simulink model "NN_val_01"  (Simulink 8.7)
settings: Solver=ode45  StartTime=0.0  StopTime=1000  RelTol=1e-3
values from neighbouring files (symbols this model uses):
  Ts = 0.05    [init_model.m]
libraries: neural x26

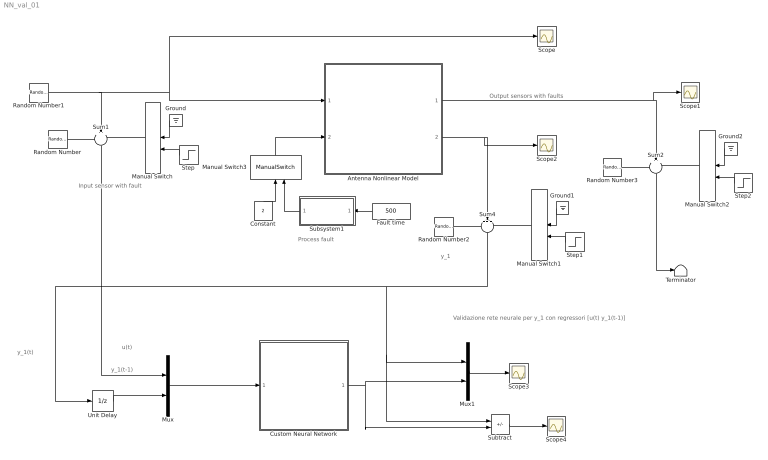
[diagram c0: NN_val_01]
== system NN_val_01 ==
  note: Validazione rete neurale per y_1 con regressori [u(t) y_1(t-1)]
  note: y_1(t)
  note: y_1(t-1)
  note: y_1
  note: u(t)
  note: Output sensors with faults
  note: Process fault
  note: Input sensor with fault
  Antenna Nonlinear Model : Subsystem
  Constant : Constant  Value=2
  Custom Neural Network : Subsystem
  Fault time : Constant  Value=500
  Ground : Ground
  Ground1 : Ground
  Ground2 : Ground
  Manual Switch{,1..3} (4 alike) : ManualSwitch
  Mux : Mux  Inputs=2
  Mux1 : Mux  Inputs=2
  Random Number : RandomNumber  Variance=0.0001  Seed=1  SampleTime=Ts
  Random Number1 : RandomNumber  Variance=0.1  SampleTime=10
  Random Number2 : RandomNumber  Variance=0.00001  Seed=2  SampleTime=Ts
  Random Number3 : RandomNumber  Variance=0.00001  Seed=3  SampleTime=Ts
  Scope{,1..4} (5 alike) : Scope
  Step : Step  Time=500  SampleTime=0
  Step1 : Step  Time=500  SampleTime=0
  Step2 : Step  Time=500  SampleTime=0
  Subsystem1 : Subsystem
  Subtract : Sum  Inputs=+-
  Sum1 : Sum  Inputs=+++  SaturateOnIntegerOverflow=on
  Sum2 : Sum  Inputs=+++  SaturateOnIntegerOverflow=on
  Sum4 : Sum  Inputs=+++  SaturateOnIntegerOverflow=on
  Terminator : Terminator
  Unit Delay : UnitDelay  SampleTime=Ts  HasFrameUpgradeWarning=on
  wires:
  Random Number1/1 -> Scope/1, Antenna Nonlinear Model/1(force), Sum1/2
  Random Number/1 -> Sum1/1
  Manual Switch/1 -> Sum1/3
  Sum1/1 -> Mux/1
  Ground/1 -> Manual Switch/1
  Step/1 -> Manual Switch/2
  Random Number2/1 -> Sum4/1
  Ground1/1 -> Manual Switch1/1
  Manual Switch1/1 -> Sum4/3
  Step1/1 -> Manual Switch1/2
  Antenna Nonlinear Model/2(velocity) -> Sum4/2, Scope2/1
  Random Number3/1 -> Sum2/1
  Ground2/1 -> Manual Switch2/1
  Manual Switch2/1 -> Sum2/3
  Step2/1 -> Manual Switch2/2
  Antenna Nonlinear Model/1(angle) -> Sum2/2, Scope1/1
  Sum2/1 -> Terminator/1
  Fault time/1 -> Subsystem1/1(Fault time)
  Subsystem1/1(Fault) -> Manual Switch3/2
  Manual Switch3/1 -> Antenna Nonlinear Model/2(drag)
  Constant/1 -> Manual Switch3/1
  Mux/1 -> Custom Neural Network/1(Input)
  Sum4/1 -> Subtract/1, Mux1/1, Unit Delay/1
  Unit Delay/1 -> Mux/2
  Custom Neural Network/1(Output) -> Subtract/2, Mux1/2
  Mux1/1 -> Scope3/1
  Subtract/1 -> Scope4/1

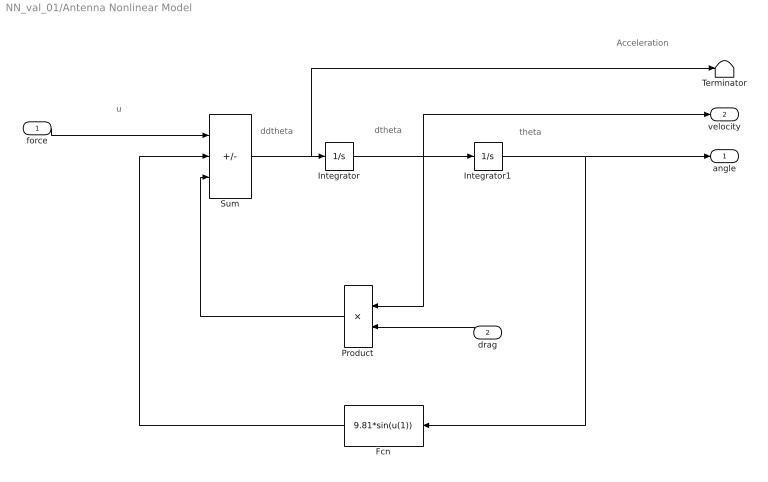
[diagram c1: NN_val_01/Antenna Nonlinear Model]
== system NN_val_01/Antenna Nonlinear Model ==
  note: Acceleration
  note: ddtheta
  note: dtheta
  note: theta
  note: u
  force : Inport
  drag : Inport  Port=2
  Fcn : Fcn  Expr=9.81*sin(u(1))
  Integrator : Integrator
  Integrator1 : Integrator  InitialCondition=(pi/180)*90
  Product : Product
  Sum : Sum  Inputs=+--  SaturateOnIntegerOverflow=on
  Terminator : Terminator
  angle : Outport
  velocity : Outport  Port=2
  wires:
  Sum/1 -> Terminator/1, Integrator/1
  Integrator/1 -> Product/1, Integrator1/1, velocity/1
  Integrator1/1 -> angle/1, Fcn/1
  Fcn/1 -> Sum/2
  Product/1 -> Sum/3
  force/1 -> Sum/1
  drag/1 -> Product/2

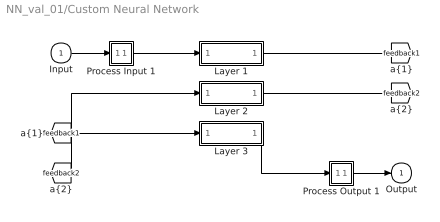
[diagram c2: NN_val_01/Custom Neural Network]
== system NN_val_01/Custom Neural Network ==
  Input : Inport  PortDimensions=2  SampleTime=0.05
  Layer 1 : Subsystem
  Layer 2 : Subsystem
  Layer 3 : Subsystem
  Process Input 1 : Subsystem
  Process Output 1 : Subsystem
  Output : Outport  InitialOutput=0
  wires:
  Input/1 -> Process Input 1/1(x)
  Process Output 1/1(y) -> Output/1
  Process Input 1/1(p) -> Layer 1/1("p{1}")
  Layer 1/1("a{1}") -> [feedback1]
  [feedback1] -> Layer 2/1("a{1} ")
  Layer 2/1("a{2}") -> [feedback2]
  [feedback2] -> Layer 3/1("a{2} ")
  Layer 3/1("a{3}") -> Process Output 1/1(a)

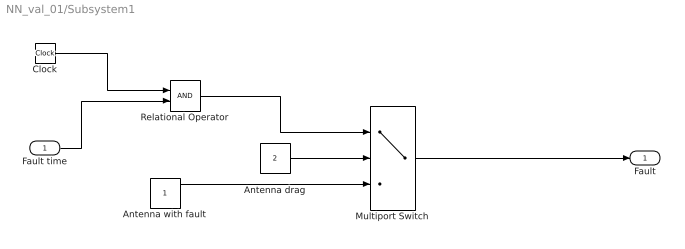
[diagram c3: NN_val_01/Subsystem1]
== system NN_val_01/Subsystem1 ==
  Fault time : Inport
  Antenna drag : Constant  Value=2
  Antenna with fault : Constant
  Clock : Clock
  Multiport Switch : MultiPortSwitch  DataPortOrder=Zero-based contiguous  Inputs=2  zeroidx=on
  Relational Operator : RelationalOperator  OutDataTypeStr=boolean
  Fault : Outport
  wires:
  Clock/1 -> Relational Operator/1
  Fault time/1 -> Relational Operator/2
  Antenna drag/1 -> Multiport Switch/2
  Relational Operator/1 -> Multiport Switch/1
  Multiport Switch/1 -> Fault/1
  Antenna with fault/1 -> Multiport Switch/3

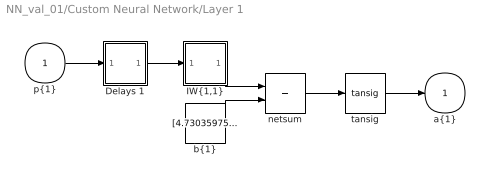
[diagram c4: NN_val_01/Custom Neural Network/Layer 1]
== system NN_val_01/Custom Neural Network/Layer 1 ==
  "p{1}" : Inport  PortDimensions=2  SampleTime=0.05
  Delays 1 : Subsystem
  "IW{1,1}" : Subsystem
  "b{1}" : Constant  Value=[4.73035975157952837122365963296033442020416259765625;1.92318223342469263315024363691918551921844482421875;0.67941730006991007950745142807136289775371551513671875;-0.8082785614923551076316243779729120433330535888671875;0.9412319551905510284228739692480303347110748291015625;-1.385422663696747491712812916375696659088134765625;4.98532785766653585568519702064804732799530029296875]
  netsum : Sum  Inputs=2  InputSameDT=on  SaturateOnIntegerOverflow=on
  tansig : neural/Transfer Functions/tansig
  "a{1}" : Outport  InitialOutput=[0;0;0;0;0;0;0]
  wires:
  "p{1}"/1 -> Delays 1/1("p{1}")
  Delays 1/1("pd{1,1}") -> "IW{1,1}"/1("pd{1,1}")
  "IW{1,1}"/1("iz{1,1}") -> netsum/1
  "b{1}"/1 -> netsum/2
  netsum/1 -> tansig/1
  tansig/1 -> "a{1}"/1

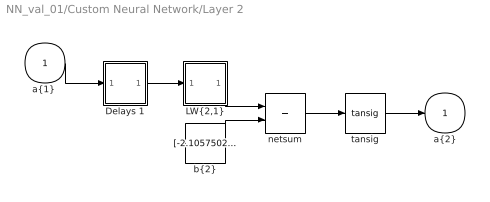
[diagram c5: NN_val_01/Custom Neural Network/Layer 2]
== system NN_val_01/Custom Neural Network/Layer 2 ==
  "a{1} " : Inport  PortDimensions=7  SampleTime=0.05
  Delays 1 : Subsystem
  "LW{2,1}" : Subsystem
  "b{2}" : Constant  Value=[-2.10575022370540665406224434264004230499267578125;-1.740826910029001250990177140920422971248626708984375;1.2556473118148903100887991968193091452121734619140625;-1.26621592229308976840229661320336163043975830078125;-0.83947473433330987990785843066987581551074981689453125;-0.6627922058413020511835611614515073597431182861328125;-0.428254180079056190333375297996099106967449188232421875;-0.1999065764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
  netsum : Sum  Inputs=2  InputSameDT=on  SaturateOnIntegerOverflow=on
  tansig : neural/Transfer Functions/tansig
  "a{2}" : Outport  InitialOutput=[0;0;0;0;0;0;0;0;0;0;0;0;0;0;0]
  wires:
  "a{1} "/1 -> Delays 1/1("p{2}")
  Delays 1/1("pd{2,1}") -> "LW{2,1}"/1("ad{2,1}")
  "LW{2,1}"/1("lz{2,1}") -> netsum/1
  "b{2}"/1 -> netsum/2
  netsum/1 -> tansig/1
  tansig/1 -> "a{2}"/1

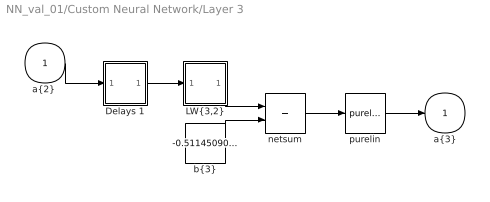
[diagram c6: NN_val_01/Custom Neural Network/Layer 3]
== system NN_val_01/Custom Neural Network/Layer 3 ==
  "a{2} " : Inport  PortDimensions=15  SampleTime=0.05
  Delays 1 : Subsystem
  "LW{3,2}" : Subsystem
  "b{3}" : Constant  Value=-0.51145090309600893530017629018402658402919769287109375
  netsum : Sum  Inputs=2  InputSameDT=on  SaturateOnIntegerOverflow=on
  purelin : neural/Transfer Functions/purelin
  "a{3}" : Outport  InitialOutput=0
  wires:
  "a{2} "/1 -> Delays 1/1("p{3}")
  Delays 1/1("pd{3,2}") -> "LW{3,2}"/1("ad{3,2}")
  "LW{3,2}"/1("lz{3,2}") -> netsum/1
  "b{3}"/1 -> netsum/2
  netsum/1 -> purelin/1
  purelin/1 -> "a{3}"/1

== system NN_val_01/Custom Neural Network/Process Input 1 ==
  x : Inport  PortDimensions=2  SampleTime=0.05
  p : Outport  PortDimensions=2  SampleTime=0.05
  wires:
  x/1 -> p/1

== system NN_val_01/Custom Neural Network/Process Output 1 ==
  a : Inport  PortDimensions=1  SampleTime=0.05
  y : Outport  PortDimensions=1  SampleTime=0.05
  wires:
  a/1 -> y/1

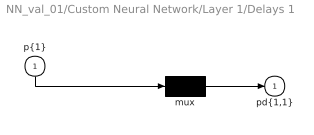
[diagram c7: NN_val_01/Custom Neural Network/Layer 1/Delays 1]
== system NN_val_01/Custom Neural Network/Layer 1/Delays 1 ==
  "p{1}" : Inport  PortDimensions=2  SampleTime=0.05
  mux : Mux  Inputs=1
  "pd{1,1}" : Outport
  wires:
  "p{1}"/1 -> mux/1
  mux/1 -> "pd{1,1}"/1

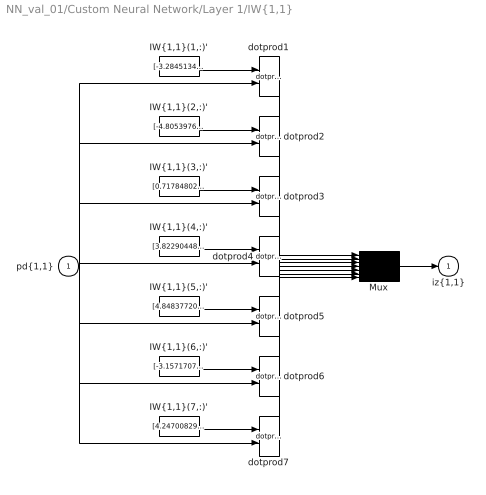
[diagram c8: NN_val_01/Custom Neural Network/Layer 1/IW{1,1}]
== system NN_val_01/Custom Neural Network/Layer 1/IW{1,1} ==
  "pd{1,1}" : Inport  PortDimensions=2  SampleTime=0.05
  "IW{1,1}(1,:)'" : Constant  Value=[-3.28451341394441076459997930214740335941314697265625;1.51253223920159829418707886361517012119293212890625]
  "IW{1,1}(2,:)'" : Constant  Value=[-4.8053976456978002573805497377179563045501708984375;-0.2265032205568367762449355495846248231828212738037109375]
  "IW{1,1}(3,:)'" : Constant  Value=[0.71784802946217818320207015858613885939121246337890625;1.456825343686549700805699103511869907379150390625]
  "IW{1,1}(4,:)'" : Constant  Value=[3.822904484041890871282021180377341806888580322265625;-1.11503162371019204357480703038163483142852783203125]
  "IW{1,1}(5,:)'" : Constant  Value=[4.848377202356548565376215265132486820220947265625;-0.284036485298596985682451077082077972590923309326171875]
  "IW{1,1}(6,:)'" : Constant  Value=[-3.1571707469550762681365085882134735584259033203125;1.4611354281525488207904572846018709242343902587890625]
  "IW{1,1}(7,:)'" : Constant  Value=[4.24700829526018086568228682153858244419097900390625;1.0876835316192134950341596777434460818767547607421875]
  Mux : Mux  Inputs=7
  dotprod{1..7} (7 alike) : neural/Weight Functions/dotprod
  "iz{1,1}" : Outport
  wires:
  "IW{1,1}(1,:)'"/1 -> dotprod1/1
  "pd{1,1}"/1 -> dotprod1/2, dotprod2/2, dotprod3/2, dotprod4/2, dotprod5/2, dotprod6/2, dotprod7/2
  dotprod1/1 -> Mux/1
  "IW{1,1}(2,:)'"/1 -> dotprod2/1
  dotprod2/1 -> Mux/2
  "IW{1,1}(3,:)'"/1 -> dotprod3/1
  dotprod3/1 -> Mux/3
  "IW{1,1}(4,:)'"/1 -> dotprod4/1
  dotprod4/1 -> Mux/4
  "IW{1,1}(5,:)'"/1 -> dotprod5/1
  dotprod5/1 -> Mux/5
  "IW{1,1}(6,:)'"/1 -> dotprod6/1
  dotprod6/1 -> Mux/6
  "IW{1,1}(7,:)'"/1 -> dotprod7/1
  dotprod7/1 -> Mux/7
  Mux/1 -> "iz{1,1}"/1

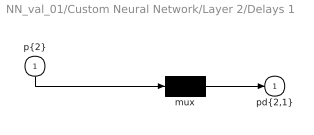
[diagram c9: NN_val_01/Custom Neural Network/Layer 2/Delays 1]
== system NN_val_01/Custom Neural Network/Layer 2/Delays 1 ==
  "p{2}" : Inport  PortDimensions=7  SampleTime=0.05
  mux : Mux  Inputs=1
  "pd{2,1}" : Outport
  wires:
  "p{2}"/1 -> mux/1
  mux/1 -> "pd{2,1}"/1

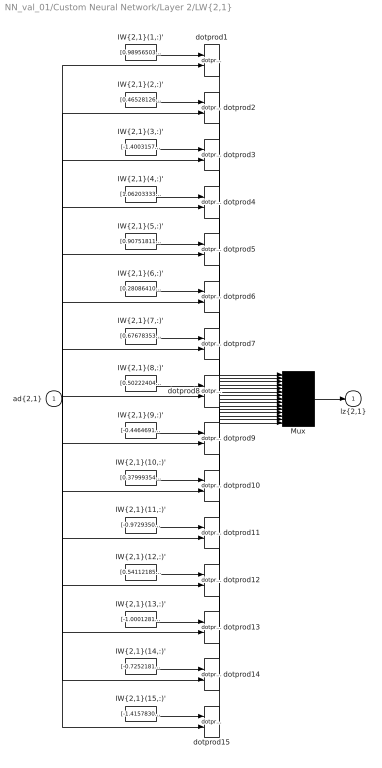
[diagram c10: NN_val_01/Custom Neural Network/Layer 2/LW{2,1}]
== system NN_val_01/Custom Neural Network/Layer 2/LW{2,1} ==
  "ad{2,1}" : Inport  PortDimensions=7  SampleTime=0.05
  "IW{2,1}(1,:)'" : Constant  Value=[0.98956503373087356667525682496489025652408599853515625;-0.82743502299202009719891748318332247436046600341796875;0.48935782268784688842089281024527736008167266845703125;0.837312553038428664109460441977716982364654541015625;-0.0999561134062968703606344433865160681307315826416015625;1.089217252024122561948615839355625212192535400390625;0.5016509412320913074978534496040083467960357666015625]
  "IW{2,1}(10,:)'" : Constant  Value=[0.37999354486878444969732981917331926524639129638671875;0.92516513421315205167871908997767604887485504150390625;-0.1307513017368535923612427041007322259247303009033203125;-0.8172231221952639401706619537435472011566162109375;-0.5678355053515049544188286745338700711727142333984375;0.1753347628075520858725866446548025123775005340576171875;-1.5465856919374909583808630486601032316684722900390625]
  "IW{2,1}(11,:)'" : Constant  Value=[-0.9729350167826316120311958002275787293910980224609375;-0.6476526715209367512926519339089281857013702392578125;-0.8623074234873244758858845671056769788265228271484375;1.07549563190858865624477402889169752597808837890625;0.1291933319203242280792665042099542915821075439453125;-0.85283803761653687036670135057647712528705596923828125;-0.2019058137223223303724495281130657531321048736572265625]
  "IW{2,1}(12,:)'" : Constant  Value=[0.5411218507500124008657849117298610508441925048828125;-0.0387980585641802544483169867817196063697338104248046875;0.421188234032296049402788185034296475350856781005859375;-0.33533087230847236082098561382736079394817352294921875;-1.073275650045232953999629899044521152973175048828125;0.20126104524410326490624356665648519992828369140625;-1.2545990277794099032604435706161893904209136962890625]
  "IW{2,1}(13,:)'" : Constant  Value=[-1.0001281330868803109979126020334661006927490234375;-0.248730783605606908803764554249937646090984344482421875;-0.517468880286684917990669418941251933574676513671875;-0.6791337962692847174395183174056001007556915283203125;-0.82969905569269375433805180364288389682769775390625;-0.80832160246701556527426646425737999379634857177734375;0.92476912049613113619983550961478613317012786865234375]
  "IW{2,1}(14,:)'" : Constant  Value=[-0.7252181362598946190445303727756254374980926513671875;0.474067733246017919412906849174760282039642333984375;0.0194129198205291557399743140877035330049693584442138671875;-0.806853469904190934158805248443968594074249267578125;0.10109242321179533197206268368972814641892910003662109375;0.497658068712021506296849793216097168624401092529296875;-1.6083532095082928581319947625161148607730865478515625]
  "IW{2,1}(15,:)'" : Constant  Value=[-1.4157830174914660670282273713382892310619354248046875;0.6312873575596233965967485346482135355472564697265625;0.50075104346758358975222336084698326885700225830078125;0.39369584753206343652465193372336216270923614501953125;0.824032181405560226750139918294735252857208251953125;0.54292108861951204890061717378557659685611724853515625;0.815480223547609739398467354476451873779296875]
  "IW{2,1}(2,:)'" : Constant  Value=[0.4652812627322584493327894961112178862094879150390625;0.8626500184084999744982269476167857646942138671875;-0.95185560342279351697669653731281869113445281982421875;1.2740087810297058279473958464222960174083709716796875;-0.48546229856707590055719947486068122088909149169921875;-1.007318585156324441953756831935606896877288818359375;-0.11690167685712993250746194462408311665058135986328125]
  "IW{2,1}(3,:)'" : Constant  Value=[-1.4003157936261576566039366298355162143707275390625;0.37223773656880598803553539255517534911632537841796875;-0.241725222047739218833584118328872136771678924560546875;0.5126417745003946091486568548134528100490570068359375;0.7280217719484676219821039921953342854976654052734375;0.2224642518789156919734040229741367511451244354248046875;-1.3409115495849650567805610990035347640514373779296875]
  "IW{2,1}(4,:)'" : Constant  Value=[1.062033337230853025090482333325780928134918212890625;-0.56867718055479576921840134673402644693851470947265625;0.458492053317244074861491753836162388324737548828125;-1.156192751944626007087890684488229453563690185546875;0.20570381960045602820486010386957786977291107177734375;-0.03781439072945809443115905423837830312550067901611328125;-0.99122707823458344744693704342353157699108123779296875]
  "IW{2,1}(5,:)'" : Constant  Value=[0.9075181152564397724091804775525815784931182861328125;0.8282789530443555037209080182947218418121337890625;-0.64541888475319364459892312879674136638641357421875;-0.62343684413991951043243489039014093577861785888671875;0.1732110715523846600216728575105662457644939422607421875;-1.1055804232581964985371314469375647604465484619140625;0.8883984542893335056845671715564094483852386474609375]
  "IW{2,1}(6,:)'" : Constant  Value=[0.280864103368938911042818062924197874963283538818359375;-1.1583458724432755815314521896652877330780029296875;-1.0093975528026513099888461511000059545040130615234375;-0.361976425619868091843045476707629859447479248046875;0.94712182610113682112995547868194989860057830810546875;-0.2928918106963351863925026918877847492694854736328125;-0.88870695446817971063779850737773813307285308837890625]
  "IW{2,1}(7,:)'" : Constant  Value=[0.67678353031291027530613746421295218169689178466796875;-0.343292778479579341333050024331896565854549407958984375;0.0004629665148357174457582896565099872532300651073455810546875;1.15948538521118127420095333945937454700469970703125;-0.53265072391484913350012675437028519809246063232421875;-1.091646998042858474065042173606343567371368408203125;0.845358357965475537554311813437379896640777587890625]
  "IW{2,1}(8,:)'" : Constant  Value=[0.50222404808635501272107148906798101961612701416015625;-0.37776398974984015666223058360628783702850341796875;0.83359979420529295435215999532374553382396697998046875;-0.59812352290377013286359897392685525119304656982421875;0.435099822256792945207592993028811179101467132568359375;0.731584888891451345926952853915281593799591064453125;-0.1699034157718363469147249134039157070219516754150390625]
  "IW{2,1}(9,:)'" : Constant  Value=[-0.446469159738944354476331000114441849291324615478515625;0.5386312734142004732262876132153905928134918212890625;-0.687930890293383168199170540901832282543182373046875;0.9826638712603388281507932333624921739101409912109375;0.49379960776870246430547695126733742654323577880859375;-0.2167146710170031187470129907524096779525279998779296875;1.251953090175079719159612068324349820613861083984375]
  Mux : Mux  Inputs=15
  dotprod{1..15} (15 alike) : neural/Weight Functions/dotprod
  "lz{2,1}" : Outport
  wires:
  "IW{2,1}(1,:)'"/1 -> dotprod1/1
  "ad{2,1}"/1 -> dotprod1/2, dotprod2/2, dotprod3/2, dotprod4/2, dotprod5/2, dotprod6/2, dotprod7/2, dotprod8/2, dotprod9/2, dotprod10/2, dotprod11/2, dotprod12/2, dotprod13/2, dotprod14/2, dotprod15/2
  dotprod1/1 -> Mux/1
  "IW{2,1}(2,:)'"/1 -> dotprod2/1
  dotprod2/1 -> Mux/2
  "IW{2,1}(3,:)'"/1 -> dotprod3/1
  dotprod3/1 -> Mux/3
  "IW{2,1}(4,:)'"/1 -> dotprod4/1
  dotprod4/1 -> Mux/4
  "IW{2,1}(5,:)'"/1 -> dotprod5/1
  dotprod5/1 -> Mux/5
  "IW{2,1}(6,:)'"/1 -> dotprod6/1
  dotprod6/1 -> Mux/6
  "IW{2,1}(7,:)'"/1 -> dotprod7/1
  dotprod7/1 -> Mux/7
  "IW{2,1}(8,:)'"/1 -> dotprod8/1
  dotprod8/1 -> Mux/8
  "IW{2,1}(9,:)'"/1 -> dotprod9/1
  dotprod9/1 -> Mux/9
  "IW{2,1}(10,:)'"/1 -> dotprod10/1
  dotprod10/1 -> Mux/10
  "IW{2,1}(11,:)'"/1 -> dotprod11/1
  dotprod11/1 -> Mux/11
  "IW{2,1}(12,:)'"/1 -> dotprod12/1
  dotprod12/1 -> Mux/12
  "IW{2,1}(13,:)'"/1 -> dotprod13/1
  dotprod13/1 -> Mux/13
  "IW{2,1}(14,:)'"/1 -> dotprod14/1
  dotprod14/1 -> Mux/14
  "IW{2,1}(15,:)'"/1 -> dotprod15/1
  dotprod15/1 -> Mux/15
  Mux/1 -> "lz{2,1}"/1

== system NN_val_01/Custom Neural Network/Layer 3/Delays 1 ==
  "p{3}" : Inport  PortDimensions=15  SampleTime=0.05
  mux : Mux  Inputs=1
  "pd{3,2}" : Outport
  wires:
  "p{3}"/1 -> mux/1
  mux/1 -> "pd{3,2}"/1

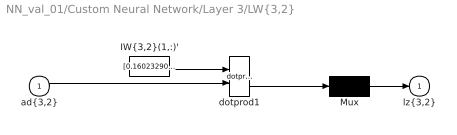
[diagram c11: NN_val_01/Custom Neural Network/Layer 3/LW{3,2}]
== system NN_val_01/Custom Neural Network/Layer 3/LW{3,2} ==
  "ad{3,2}" : Inport  PortDimensions=15  SampleTime=0.05
  "IW{3,2}(1,:)'" : Constant  Value=[0.16023290154776781424317277924274094402790069580078125;0.433121017432581412176517687839805148541927337646484375;-0.4461323362559974636809556614025495946407318115234375;0.2188257889665365107934036359438323415815830230712890625;-0.11178384444804766173486854086149833165109157562255859375;0.28892835116905646319906963981338776648044586181640625;0.203596558882588291039539285520731937140226364135742187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
  Mux : Mux  Inputs=1
  dotprod1 : neural/Weight Functions/dotprod
  "lz{3,2}" : Outport
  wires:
  "IW{3,2}(1,:)'"/1 -> dotprod1/1
  "ad{3,2}"/1 -> dotprod1/2
  dotprod1/1 -> Mux/1
  Mux/1 -> "lz{3,2}"/1
